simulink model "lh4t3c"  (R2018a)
settings: Solver=ode45  StartTime=0.0  StopTime=1000  RelTol=1e-3  AbsTol=1e-6
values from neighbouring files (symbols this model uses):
  a = 0.01    [lh4t3_m.m]
  K = hairio    (= 1)    [lh4t3_m.m]
  x_1_0 = 5.0    (= 5)    [lh4t3_m.m]
  x_2_0 = 0.0    (= 0)    [lh4t3_m.m]
libraries: simulink x1

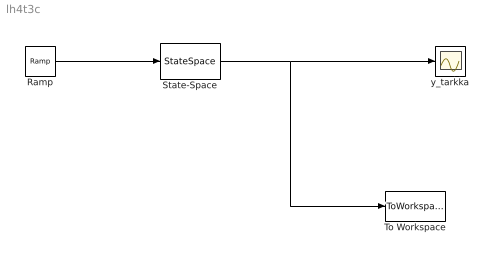
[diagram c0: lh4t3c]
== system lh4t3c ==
  Ramp : simulink/Sources/Ramp  slope=a  start=0  InitialOutput=K
  State-Space : StateSpace  A=[-0.001 0; 0 -1000]  B=[0.001; 1000]  C=[1 1]  D=0  InitialCondition=[x_1_0 x_2_0]
  To Workspace : ToWorkspace  VariableName=y_tarkka  SampleTime=-1
  y_tarkka : Scope
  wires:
  Ramp/1 -> State-Space/1
  State-Space/1 -> To Workspace/1, y_tarkka/1
